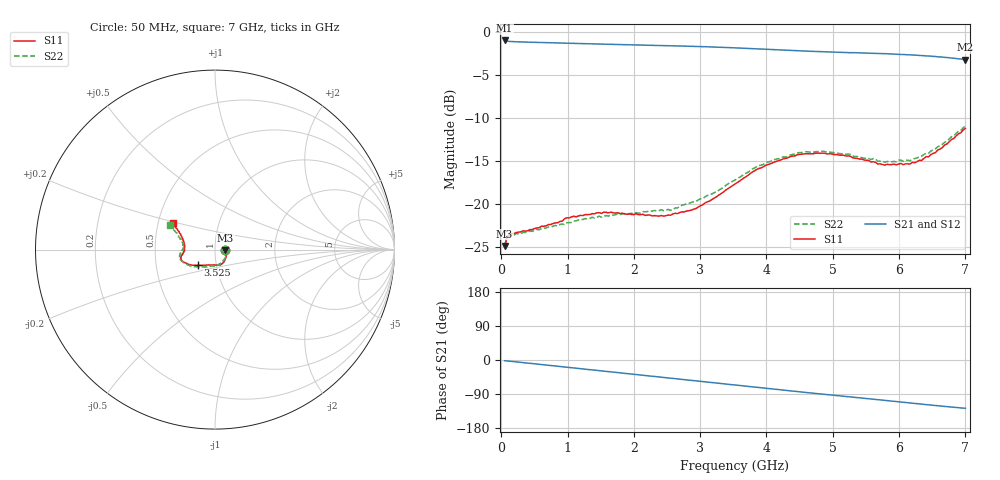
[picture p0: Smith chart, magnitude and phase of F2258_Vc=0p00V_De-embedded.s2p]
! Integrated Device Technology
! Corporate Headquarters
! 6024 Silver Creek Valley Road
! San Jose, CA 95138  USA
! Phone:  1-408-284-8200
! Toll Free:  1-800-223-1366
! Webpage:  http://www.idt.com/
! Timing and RF Division
! 515 Groton Road, Suite 102
! Westford, MA 01886-6024
! Device:  F2258
! Description: Voltage Variable RF Attenuator
! Frequency:  50.0 -  6000.00 MHz
! Package:  3x3 mm Thin QFN Plastic Package: 16 pin
! Ports:  2 RF, 2 DC
!  Pin  1  = NC
!  Pin  2  = NC
!  Pin  3  = RF2  = Port 2
!  Pin  4  = GND
!  Pin  5  = Vdd
!  Pin  6  = NC
!  Pin  7  = VCTRL
!  Pin  8  = NC
!  Pin  9  = GND
!  Pin 10  = RF1  = Port 1
!  Pin 11  = NC
!  Pin 12  = NC
!  Pin 13  = NC
!  Pin 14  = NC
!  Pin 15  = NC
!  Pin 16  = NC
! Vcntrl:  0.000 Volts
! Vdd:  +3.300 Volts
! Current:  1.076 mA
! Data:  The device was measured on a the F2258 evaluation board which has
!  individual transmission lines to the RF pins.  Data was collected
!  using a calibrated network analyzer.  The evaluation board was
!  de-embedded using a TRL calibration technique.
!  The reference plane is the edge of the package pin.
! Misc:  SN 10
!  Action Tracker AT0285
! Date Measured:  2014-12-10
! Date:  2016-01-13  MJV
! Note:
!  Integrated Device Technology supplies this data as a sample of measured
!  data at the package pin for this product.  Your particular data for this
!  product may vary.
!  Data was taken at 25 degrees C.
!  Integrated Device Technology reserves the right to change this data at anytime.
!Freq_(GHz)  S11M_(dB)  S11P_(deg)  S21M_(dB)  S21P_(deg)  S12M_(dB)  S12P_(deg)  S22M_(dB)  S22P_(deg)
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# GHz S dB R 50
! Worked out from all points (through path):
!   201 points, 50 MHz to 7 GHz, reference 50 ohm
!   highest |S21| = -0.96 dB at 50 MHz (marker M1); lowest = -3.2 dB at 7 GHz (marker M2)
!   group delay of S21, straight-line fit = 50.5 ps
!   lowest |S11| = -24.9 dB at 50 MHz (marker M3), VSWR 1.12, Z = 56 - j0.391 ohm
!   |S11| at or under -10 dB: start of sweep to end of sweep
!   |S22| runs from -24.9 to -10.9 dB; largest |S21 - S12| = 0.00042
!   S11 on the Smith chart (normalised r, x): 50 MHz: 1.12, -0.01; 3.525 GHz: 0.81, -0.14; 7 GHz: 0.60, +0.19
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0.05  -24.88 -3.5  -0.96 -1.9  -0.96 -1.9  -24.91 -3.0
0.08475  -23.91 -6.0  -1.03 -2.4  -1.03 -2.5  -23.98 -5.5
0.15425  -23.42 -9.3  -1.08 -3.6  -1.08 -3.6  -23.60 -9.4
0.71025  -22.40 -37.2  -1.22 -14.1  -1.22 -14.1  -22.69 -38.6
0.91875  -22.00 -47.0  -1.26 -18.0  -1.26 -18.0  -22.33 -50.4
0.98825  -21.60 -51.0  -1.27 -19.3  -1.27 -19.3  -22.18 -54.8
1.2315  -21.35 -59.3  -1.32 -23.8  -1.32 -23.8  -21.80 -63.8
1.6485  -20.94 -71.0  -1.41 -31.4  -1.41 -31.4  -21.31 -76.7
2.37825  -21.42 -92.4  -1.54 -44.7  -1.54 -44.7  -20.77 -94.3
2.552  -21.31 -98.4  -1.57 -48.0  -1.57 -48.0  -20.74 -99.6
2.93425  -20.53 -115.1  -1.65 -55.1  -1.65 -55.1  -19.73 -112.9
3.525  -17.69 -137.8  -1.82 -66.2  -1.82 -66.2  -17.21 -135.6
4.0115  -15.43 -151.3  -2.00 -75.2  -2.00 -75.2  -15.12 -151.0
4.46325  -14.28 -159.8  -2.16 -83.4  -2.16 -83.4  -14.07 -162.0
4.7065  -14.14 -163.0  -2.23 -87.7  -2.23 -87.6  -13.96 -166.3
5.2625  -14.42 -170.0  -2.38 -97.3  -2.38 -97.3  -14.21 -174.2
5.6795  -15.35 -176.8  -2.47 -104.6  -2.47 -104.6  -15.03 -179.6
5.85325  -15.42 179.0  -2.52 -107.8  -2.52 -107.8  -15.07 175.8
6.166  -15.34 171.2  -2.63 -113.4  -2.63 -113.3  -14.97 169.8
6.33975  -14.93 164.9  -2.71 -116.5  -2.71 -116.5  -14.43 165.5
6.722  -13.01 153.3  -2.94 -123.1  -2.94 -123.1  -12.71 156.4
7  -11.20 147.9  -3.19 -127.4  -3.19 -127.4  -10.92 151.5
